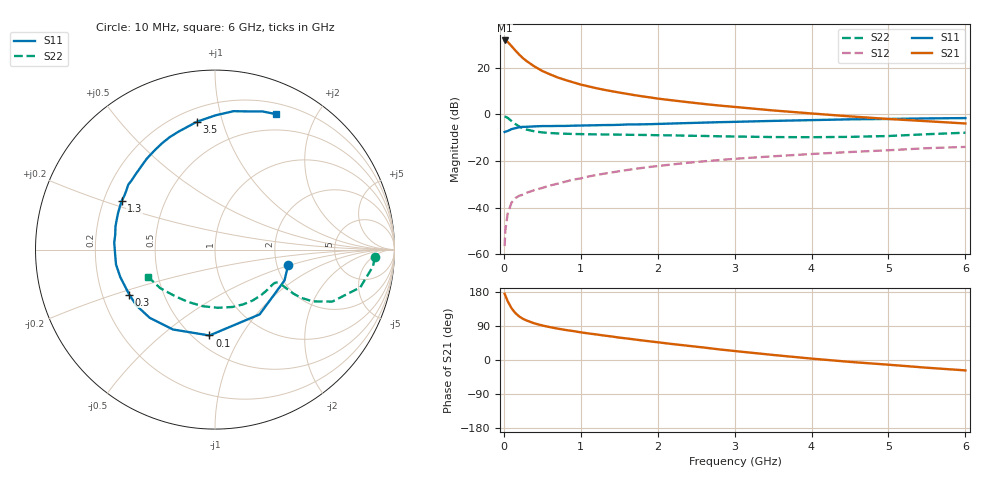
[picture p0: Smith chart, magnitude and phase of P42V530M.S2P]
! SIEMENS Small Signal Semiconductors
! BFP182
! Si NPN RF Bipolar Junction Transistor in SOT143
! VCE = 2.5 V  IC = 30 mA
! Common Emitter S-Parameters:  March  1996
# GHz  S  MA  R  50
!  f  S11  S21  S12  S22
! GHz  MAG  ANG  MAG  ANG  MAG  ANG  MAG  ANG
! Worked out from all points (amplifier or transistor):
!   36 points, 10 MHz to 6 GHz, reference 50 ohm
!   highest |S21| = 31.6 dB at 10 MHz (marker M1)
!   |S21| within 3 dB of that: start of sweep to 115 MHz
!   unconditionally stable (mu >= 1): start of sweep to 14.92 MHz; 372.3 MHz to end of sweep
!   at 250 MHz: K = 0.81, MSG = 29.2 dB, |S12| = -34.4 dB
!   at 1.4 GHz: K = 1.48, MAG = 13.3 dB, |S12| = -24.9 dB
!   at 6 GHz: K = 1.06, MAG = 3.5 dB, |S12| = -14.0 dB
!   S11 on the Smith chart (normalised r, x): 10 MHz: 2.31, -0.48; 100 MHz: 0.60, -0.74; 300 MHz: 0.32, -0.22; 1.3 GHz: 0.28, +0.23; 3.5 GHz: 0.28, +0.83; 6 GHz: 0.31, +1.50
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0.01  0.4165 -11.8  37.95 174.8  0.0015 78.3  0.8915 -2.7
0.02  0.4237 -24.0  37.91 169.9  0.0033 74.6  0.8855 -6.0
0.05  0.4383 -55.4  35.29 155.2  0.0075 73.5  0.8362 -14.6
0.1  0.4795 -93.7  28.63 136.6  0.0128 57.6  0.7148 -23.9
0.15  0.5028 -117.7  23.16 123.8  0.016 51.9  0.6169 -27.9
0.2  0.526 -133.7  18.93 114.9  0.018 50.0  0.5466 -29.3
0.25  0.5375 -144.6  15.78 108.5  0.019 49.0  0.4988 -29.3
0.3  0.5395 -152.3  13.58 103.9  0.0209 49.0  0.4677 -28.8
0.4  0.5495 -163.8  10.49 96.5  0.0239 50.0  0.4292 -28.0
0.5  0.5578 -171.5  8.437 91.1  0.0265 52.3  0.4082 -27.5
0.6  0.5575 -178.5  7.148 86.7  0.0298 53.9  0.396 -27.7
0.7  0.5627 176.0  6.119 82.8  0.0327 56.0  0.3883 -28.1
0.8  0.5621 171.4  5.406 79.3  0.0361 56.6  0.3826 -29.0
1.1  0.5772 159.3  3.951 70.1  0.0466 58.0  0.3729 -32.7
1.3  0.5864 152.6  3.341 64.6  0.0534 57.7  0.3686 -35.9
1.7  0.6041 139.9  2.559 54.2  0.0675 56.4  0.3621 -43.1
2.2  0.6338 126.7  1.974 41.9  0.0847 53.0  0.3529 -53.5
2.8  0.6756 111.9  1.535 28.0  0.1046 48.0  0.3371 -67.9
3.5  0.7201 97.9  1.206 13.3  0.1259 41.5  0.3246 -87.2
4.5  0.778 82.4  0.9 -5.0  0.1554 32.6  0.3279 -117.2
5.5  0.8142 71.0  0.709 -20.4  0.1875 23.6  0.3737 -145.1
6  0.8274 65.8  0.634 -27.4  0.2 18.2  0.4022 -157.8
